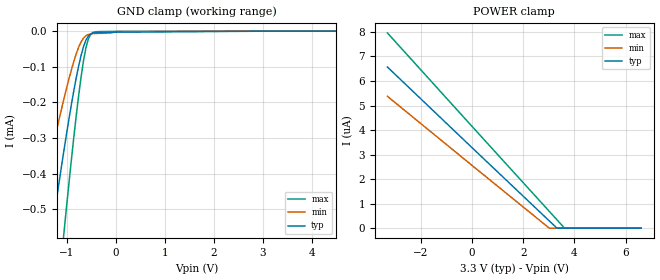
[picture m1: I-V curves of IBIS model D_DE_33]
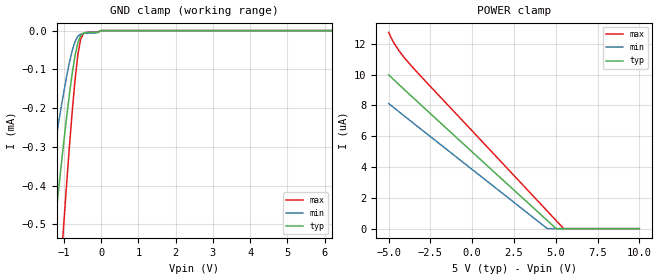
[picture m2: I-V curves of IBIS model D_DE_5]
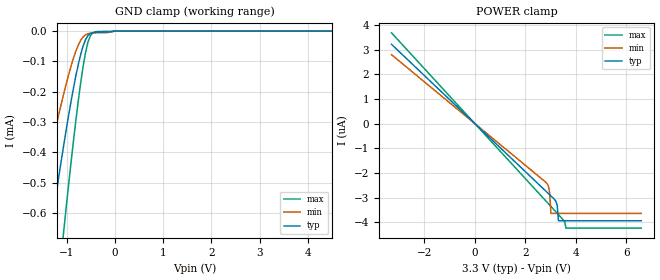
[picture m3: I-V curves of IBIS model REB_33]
| Texas Instruments Incorporated
| Isolated 5V RS-485 Transceiver with Integrated Transformer Driver
| Bit Rate of 20 Mbps
| Marketing part#   Voltage Range   Package-type   #pins/pkg drawing
| ISO3086TDW   3.0V - 5.5V   16-SOIC   16-pin DW
| ISO3086TDWR   3.0V - 5.5V   16-SOIC   16-pin DW
[IBIS Ver]   4.0
[File name]   iso3086t.ibs
[File Rev]   1.0
[Date]   02/28/2011
[Source]   Model built from TISPICE simulations at:
   Texas Instruments Incorporated.
   Analog-eLab, HPA
   12500 TI Blvd
   Dallas, TX -75243
   For Support e-mail: elab_scm_ibis@list.ti.com
[Notes]   Revision History
   Rev 1.0: 02/28/2011
   - Model based on simulations from TIspice
   - HVD3086 models borrowed from v1.0 IBIS model of iso3086e.ibs
   - ccomp values are based on PVT conditions although listed
   in numerical order, please review ccomp comments below under
   respective [Model]
   - Updated all hvd3086 models with timing, load and threshold parameters
   - Updated R_5 and R_33 model to point to correct 5V data
   - Updated series1M_* models with 1e6 resistance for all corners
   - Updated ccomp for REB_* models
   - Removed *_33 models for A/B and Y/Z as they work only on VCC2
   5.0V supply
[Disclaimer] This product is designed as an aid for customers of Texas
   Instruments.
   No warranties, either expressed or implied, with respect
   to this third party software (if any) or with respect to
   its fitness for any particular purpose is claimed by Texas
   Instruments or the author. The software (if any) is provided
   solely on an "as is" basis. The entire risk as to its quality
   and performance is with the customer
[Copyright]   (C)Copyright 2011 Texas Instruments Incorporated.
   All rights reserved.
|   Component iso3086tdw
[Component]   iso3086tdw
[Manufacturer]  Texas Instruments Incorporated
[Package]   |16-pin SOIC DW package
|   typ   min   max
R_pkg   0.05349   0.00236   0.10896
L_pkg   2.09279nH   1.06722nH   2.8015nH
C_pkg   0.56578pF   0.3807pF   0.8055pF
[Pin] signal_name   model_name   R_pin   L_pin   C_pin
1   D1   NC   0.03021   2.53109nH   0.80432pF
2   D2   NC   0.0289   1.84883nH   0.67747pF
3   GND1   GND   0.0134   1.3317nH   1.43035pF
4   VCC1   POWER   0.01669   1.09719nH   0.54298pF
5   R   R   0.02236   1.46006nH   0.62553pF
6   REB   REB   0.02303   1.06722nH   0.45571pF
7   DE   D_DE   0.03933   1.80876nH   0.6069pF
8   D   D_DE   0.04286   2.67717nH   0.80551pF
9   GND2   GND   0.0335   3.06962nH   2.59609pF
10   NC   NC   0.07414   2.77643nH   0.65609pF
11   Y   Y_5   0.10896   2.8015nH   0.42184pF
12   Z   Z_5   0.07328   2.02632nH   0.39304pF
13   B   B_5   0.06125   1.77172nH   0.3807pF
14   A   A_5   0.08402   2.2516nH   0.39641pF
15   GND2   GND   0.00043   0.6838nH   3.08028pF
16   Vcc2   POWER   0.03202   3.25704nH   0.92513pF
[Diff_pin]   inv_pin   vdiff   tdelay_typ   tdelay_min   tdelay_max
| The A and B are Diff_pins
| The Y and Z are Diff_pins
11   12   0.2   NA   NA   NA
14   13   NA   NA   NA   NA
[series pin mapping]  pin_2   model_name
6   3   series1M   |REB
7   4   series1M   |DE
8   3   series1M   |D
[Pin Mapping]pulldown_ref pullup_ref gnd_clamp_ref power_clamp_ref |ext_ref
1   NC   NC  |D1
2   NC   NC  |D2
3   GNDBUS1   NC   |GND1
4   NC   PWRBUS1 |VCC1
5   GNDBUS1   PWRBUS1   NC   NC   | R
6   NC   NC   GNDBUS1   PWRBUS1  | RE_N
7   NC   NC   GNDBUS1   PWRBUS1  | DE
8   NC   NC   GNDBUS1   PWRBUS1  | D
9   GNDBUS2   NC   |GND2 to Y/Z
10   NC   NC   |NC
11   GNDBUS2   PWRBUS2   NC   NC   | Y   Diff. Out. P
12   GNDBUS2   PWRBUS2   NC   NC   | Z   Diff. Out. N
13   NC   NC   GNDBUS2   PWRBUS2  | B   Diff. Inp. N
14   NC   NC   GNDBUS2   PWRBUS2  | A   Diff. Inp. P
15   GNDBUS2   NC   |GND2 to Y/Z
16   NC   PWRBUS2  |VCC2 to Y/Z
[Model Selector] series1M
series1M_33   series1M model for 3.00V  - 3.60V
series1M_5   series1M model for 4.50V  - 5.50V
[Model Selector] D_DE
D_DE_33   D_DE Input model for 3.00V  - 3.60V
D_DE_5   D_DE Input model for 4.50V  - 5.50V
[Model Selector] REB
REB_33   REB Input model for 3.005V  - 3.60V
REB_5   REB Input model for 4.50V  - 5.50V
[Model Selector] R
R_33   R Output model for 3.00V  - 3.60V
R_5   R Output model for 4.50V  - 5.50V
|   series1M_33 Model
[Model]   series1M_33
Model_type   Series
C_comp   0pF   0pF   0pF
[Voltage Range]   3.3V   3.00V   3.6V
[Pullup Reference]   3.3V   3.00V   3.6V
|It is pullup   resistor for D and REB
|It is pulldown resistor for DE
[Temperature Range]   40   125   -40
[R series]   1e6   1e6   1e6
|   series1M_5 Model
[Model]   series1M_5
Model_type   Series
C_comp   0pF   0pF   0pF
[Voltage Range]   5V   4.5V   5.5V
[Pullup Reference]   5V   4.5V   5.5V
|It is pullup   resistor for D and REB
|It is pulldown resistor for DE
[Temperature Range]   40   125   -40
[R series]   1e6   1e6   1e6
| Models and submodels in the file (12): series1M_33 (Series), series1M_5 (Series), D_DE_33 (Input), D_DE_5 (Input), REB_33 (Input), REB_5 (Input), R_33 (3-state), R_5 (3-state), A_5 (Input), B_5 (Input), Y_5 (Output), Z_5 (Output)
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|   D_33 and DE_33 Model
[Model]   D_DE_33
Model_type   Input
Vinl   = 0.99V
Vinh   = 2.31V
|   typ   min   max
|   (nom PVT)   (Fast PVT)   (Slow PVT)
C_comp   0.25330444pF   0.25330444pF  0.25330445pF
[Model Spec]
Vinl   0.99V   0.9V   1.08V
Vinh   2.31V   2.1V   2.52V
[Voltage Range]   3.3   3.0   3.6
[Temperature Range]   40   125   -40
[Power Clamp Reference]   3.3   3.0   3.6
[GND Clamp Reference]   0   0   0
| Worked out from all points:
|   GND clamp passes 1 mA (typ) near -1.76 V on its own axis
[GND Clamp]
|   Voltage   I(typ)   I(min)   I(max)
-3.3V     -2.706mA   -1.77mA    -4.192mA
-1.658V   -902.1uA   -559.6uA   -1.442mA
-1.31V    -563.2uA   -337.7uA   -921.6uA
-1.061V   -333.8uA   -189.4uA   -565uA
-862.3mV  -168.7uA   -85.87uA   -300uA
-713.1mV  -68.72uA   -30.52uA   -129.5uA
-663.3mV  -43.98uA   -19.72uA   -83.66uA
-613.6mV  -25.51uA   -13uA      -46.93uA
-563.8mV  -13.85uA   -9.395uA   -21.91uA
-464.3mV  -5.433uA   -6.906uA   -3.589uA
0V        -2.989uA   -1.392uA   -1.01uA
6.6V      0A         0A         0A
[POWER Clamp]
|   Voltage   I(typ)   I(min)   I(max)
-3.3V     6.571uA    5.377uA    7.961uA
3.018V    295.7nA    0A         685.8nA
3.317V    0A         0A         342.9nA
3.615V    0A         0A         0A
6.6V      0A         0A         0A
|   D_5 & DE_5 Model
[Model]   D_DE_5
Model_type   Input
Vinl   = 1.5V
Vinh   = 3.5V
|   typ   min   max
|   (nom PVT)   (Slow PVT)   (Fast PVT)
C_comp   0.25330467pF   0.25330466pF   0.25330470pF
[Model Spec]
Vinl   1.5V   1.35V   1.65V
Vinh   3.5V   3.15V   3.85V
[Voltage Range]   5   4.5   5.5
[Temperature Range]   40   125   -40
[Power Clamp Reference]   5   4.5   5.5
[GND Clamp Reference]   0   0   0
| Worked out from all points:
|   GND clamp passes 1 mA (typ) near -1.75 V on its own axis
[GND Clamp]
|   Voltage   I(typ)   I(min)   I(max)
-5V       -4.809mA   -3.207mA   -7.295mA
-1.608V   -855.4uA   -527.7uA   -1.379mA
-1.307V   -562.2uA   -336.1uA   -929.7uA
-1.231V   -491uA     -289.9uA   -819.3uA
-1.08V    -352.8uA   -200.8uA   -603.1uA
-1.005V   -286.8uA   -158.7uA   -498.3uA
-854.3mV  -164.4uA   -82.63uA   -299.6uA
-703.5mV  -64.98uA   -28.46uA   -128uA
-628.1mV  -31.41uA   -14.89uA   -62.92uA
-552.8mV  -13.06uA   -9.174uA   -22.43uA
0V        0A         0A         0A
10V       0A         0A         0A
[POWER Clamp]
|   Voltage   I(typ)   I(min)   I(max)
-5V       9.993uA    8.125uA    12.75uA
-4.774V   9.756uA    7.927uA    12.23uA
-4.472V   9.446uA    7.666uA    11.69uA
-3.643V   8.608uA    6.953uA    10.57uA
4.497V    522.7nA    0A         1.135uA
5.025V    0A         0A         523.9nA
5.477V    0A         0A         0A
10V       0A         0A         0A
|   REB_33 Model
[Model]   REB_33
Model_type   Input
Vinl   = 0.99V
Vinh   = 2.31V
|   typ   min   max
|   (nom PVT)   (Slow PVT)   (Fast PVT)
C_comp   0.25330759pF  0.25330759pF  0.25330760pF
[Model Spec]
Vinl   0.99V   0.9V   1.08V
Vinh   2.31V   2.1V   2.52V
[Voltage Range]   3.3   3.0   3.6
[Temperature Range]   40   125   -40
[Power Clamp Reference]   3.3   3.0   3.6
[GND Clamp Reference]   0   0   0
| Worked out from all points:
|   GND clamp passes 1 mA (typ) near -1.63 V on its own axis
[GND Clamp]
|   Voltage   I(typ)   I(min)   I(max)
-3.3V     -3.1mA     -2.088mA   -4.612mA
-1.708V   -1.087mA   -684uA     -1.729mA
-1.658V   -1.029mA   -644uA     -1.642mA
-1.36V    -687.9uA   -413.3uA   -1.136mA
-1.31V    -633.3uA   -376.7uA   -1.053mA
-1.061V   -373uA     -204.8uA   -655.6uA
-762.8mV  -110.5uA   -46.29uA   -230.7uA
-663.3mV  -49.71uA   -19.34uA   -117.5uA
-563.8mV  -15.33uA   -8.682uA   -37.76uA
-464.3mV  -5.241uA   -6.119uA   -6.24uA
-315.1mV  -3.519uA   -5.499uA   -1.249uA
6.6V      0A         0A         0A
[POWER Clamp]
|   Voltage   I(typ)   I(min)   I(max)
-3.3V     3.211uA    2.79uA     3.676uA
2.819V    -2.743uA   -2.388uA   -3.14uA
2.919V    -2.84uA    -2.542uA   -3.251uA
2.968V    -2.888uA   -2.813uA   -3.307uA
3.018V    -2.936uA   -3.644uA   -3.362uA
3.217V    -3.153uA   -3.644uA   -3.584uA
3.267V    -3.316uA   -3.644uA   -3.639uA
3.317V    -3.942uA   -3.644uA   -3.694uA
3.565V    -3.942uA   -3.644uA   -3.994uA
3.615V    -3.942uA   -3.644uA   -4.242uA
6.6V      -3.942uA   -3.644uA   -4.242uA
